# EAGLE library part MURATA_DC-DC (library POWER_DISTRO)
UWS Series DC-CD, Thru-hole
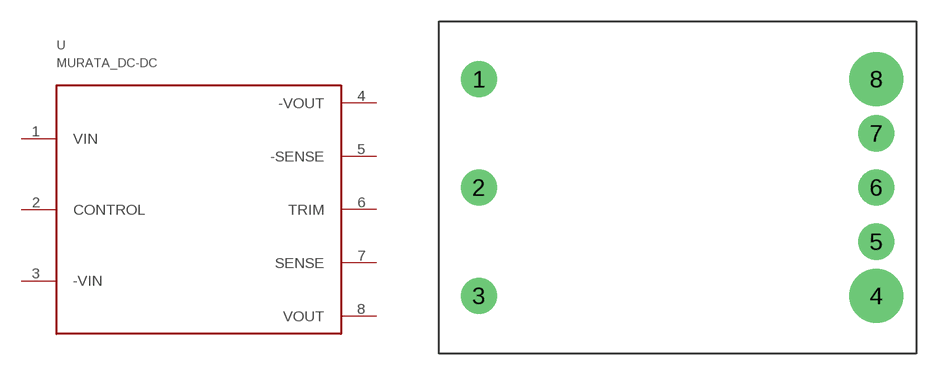
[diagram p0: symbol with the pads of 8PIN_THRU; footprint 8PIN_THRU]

Designator prefix -

## MURATA_DC-DCTHRU  [8PIN_THRU]
1  VIN
2  CONTROL
3  -VIN
4  -VOUT
5  -SENSE
6  TRIM
7  SENSE
8  VOUT

## Footprint 8PIN_THRU (pad centres in mm)
8-pin, Through-hole mount
drill 1.575 pad 2.54: 1 -13.97,7.62; 2 -13.97,0; 3 -13.97,-7.62; 5 13.97,-3.81; 6 13.97,0; 7 13.97,3.81
drill 2.134 pad 3.81: 4 13.97,-7.62; 8 13.97,7.62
